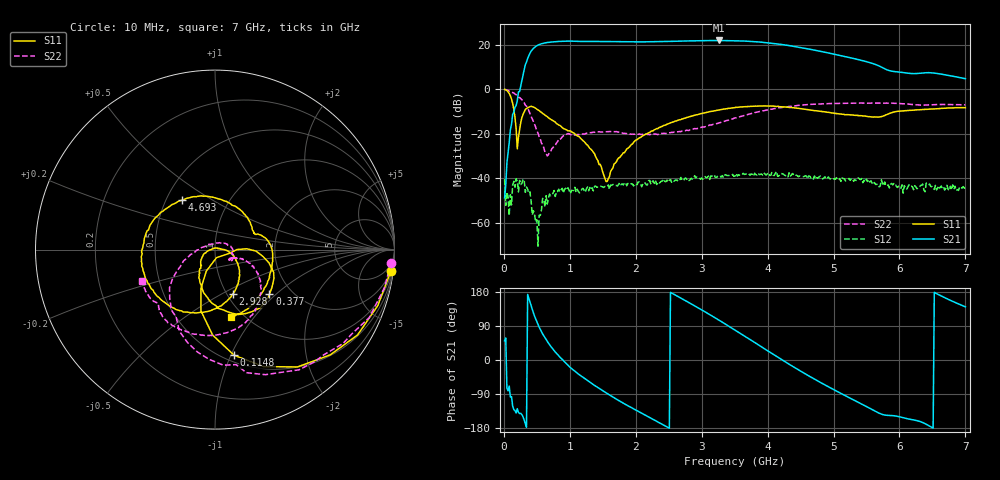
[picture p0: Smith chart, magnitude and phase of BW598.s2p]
!Agilent Technologies,N5244A,MY49441013,A.09.90.07
!Agilent N5244A: A.09.90.07
!Date: Wednesday, May 21, 2014 11:08:38
!Correction: S11(Full 2 Port with power(1,2))
!S21(Full 2 Port with power(1,2))
!S12(Full 2 Port with power(1,2))
!S22(Full 2 Port with power(1,2))
!S2P File: Measurements: S11, S21, S12, S22:
# Hz S  dB  R 50
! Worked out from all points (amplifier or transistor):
!   401 points, 10 MHz to 7 GHz, reference 50 ohm
!   highest |S21| = 21.8 dB at 3.26 GHz (marker M1)
!   |S21| within 3 dB of that: 469.1 MHz to 4.467 GHz (3.998 GHz wide, 162 % of centre)
!   unconditionally stable (mu >= 1): start of sweep to end of sweep
!   at 1.163 GHz: K = 8.45, MAG = 21.5 dB, |S12| = -46.0 dB
!   at 3.505 GHz: K = 3.09, MAG = 22.6 dB, |S12| = -39.0 dB
!   at 7 GHz: K = 37.98, MAG = 6.3 dB, |S12| = -45.6 dB
!   S11 on the Smith chart (normalised r, x): 10 MHz: 2, -17; 114.8 MHz: 0.56, -1.03; 377 MHz: 1.55, -0.91; 2.928 GHz: 1.07, -0.57; 4.693 GHz: 0.60, +0.37; 7 GHz: 0.88, -0.77
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1e7  -0.10 -6.8  -48.81 50.5  -40.44 82.9  -0.14 -4.5
1.1485e8  -4.46 -79.7  -15.77 -96.6  -51.98 133.4  -1.48 -43.9
3.07075e8  -10.20 -13.7  8.71 -158.3  -40.88 -37.2  -6.09 -113.6
3.76975e8  -8.13 -39.3  14.97 163.2  -46.73 -56.6  -9.63 -140.1
4.81825e8  -8.66 -74.4  19.15 108.3  -59.71 -57.9  -17.10 -168.4
5.86675e8  -10.96 -96.8  20.43 68.9  -49.05 57.2  -25.00 161.0
7.09e8  -13.52 -111.7  21.10 36.4  -47.90 37.4  -27.97 65.0
8.488e8  -16.35 -125.1  21.39 7.7  -46.12 16.8  -22.59 19.9
1.180825e9  -22.62 -154.2  21.37 -43.6  -44.97 10.3  -20.33 -12.2
1.425475e9  -32.08 -177.0  21.38 -73.0  -44.01 -1.6  -19.19 -23.0
1.670125e9  -33.60 19.7  21.31 -99.5  -42.72 -8.5  -19.08 -32.5
2.35165e9  -17.30 -28.5  21.30 -165.1  -42.09 -45.2  -20.22 -29.5
2.648725e9  -13.92 -47.4  21.51 166.7  -40.54 -56.3  -19.14 -23.5
2.928325e9  -11.48 -68.1  21.67 139.2  -39.44 -68.5  -17.75 -21.6
3.26035e9  -9.37 -93.8  21.83 105.2  -39.11 -80.5  -15.18 -19.1
3.505e9  -8.30 -115.3  21.71 79.1  -39.03 -93.8  -12.91 -23.1
4.046725e9  -7.57 -167.3  20.62 19.2  -38.74 -124.7  -9.05 -43.8
4.675825e9  -9.50 125.6  17.68 -47.0  -39.72 -165.3  -6.85 -74.3
4.6933e9  -9.61 123.4  17.59 -48.7  -40.44 -166.8  -6.82 -75.0
5.304925e9  -11.67 54.9  13.73 -105.4  -41.39 162.9  -6.35 -101.2
5.84665e9  -10.94 13.7  8.29 -146.2  -44.39 134.8  -6.30 -121.5
7e9  -8.31 -76.2  4.68 140.4  -45.55 87.7  -7.09 -156.6
